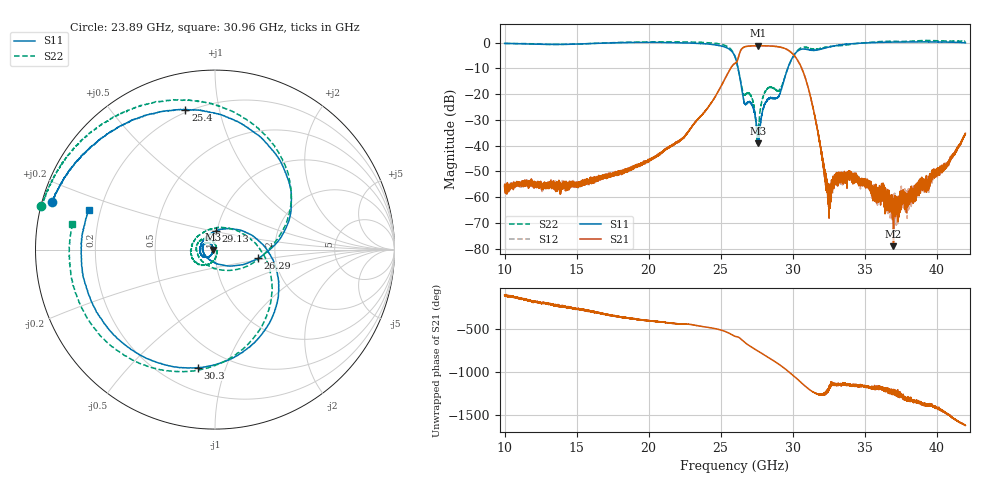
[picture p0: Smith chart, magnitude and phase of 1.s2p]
!The following data was pulled from an Agilent PNA
!This sNp file was generated from the data in the RF Test software
!NOTE:  Smoothing/Math/Corrections applied on any given trace ARE included in the data saved here
# MHz S dB R 50
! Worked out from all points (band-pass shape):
!   12801 points, 10 GHz to 42 GHz, reference 50 ohm
!   highest |S21| = -1.25 dB at 27.63 GHz (marker M1); lowest = -79.1 dB at 37.01 GHz (marker M2)
!   |S21| within 3 dB of the highest: 26.31 GHz to 29.98 GHz (3.668 GHz wide, 13 % of centre)
!   lowest |S11| = -39.2 dB at 27.63 GHz (marker M3), VSWR 1.02, Z = 48.9 - j0.0915 ohm
!   |S11| at or under -10 dB: 26.21 GHz to 29.66 GHz (3.449 GHz wide, 12.3 % of centre)
!   |S22| runs from -39.4 to 0.8 dB; largest |S21 - S12| = 0.0073
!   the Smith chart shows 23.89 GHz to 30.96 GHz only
!   S11 on the Smith chart (normalised r, x): 23.89 GHz: 0.03, +0.14; 25.4 GHz: 0.18, +0.79; 26.29 GHz: 1.62, -0.17; 29.13 GHz: 0.99, +0.21; 30.3 GHz: 0.34, -0.81; 30.96 GHz: 0.15, +0.15
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10000  -0.34 144.0  -56.36 -108.2  -56.17 -106.3  -0.36 144.1
12945  -0.73 74.5  -54.89 155.6  -55.10 153.8  -0.73 75.6
15335  -0.55 -9.8  -54.07 77.9  -54.62 84.4  -0.54 -9.2
17607.5  -0.09 -78.2  -51.10 15.2  -51.23 14.1  -0.05 -77.6
20667.5  0.03 -136.5  -43.44 -54.9  -43.69 -55.0  0.24 -135.3
23885  -0.49 163.8  -26.93 -116.1  -26.94 -116.5  -0.02 165.9
25400  -1.96 102.0  -13.01 -175.3  -13.00 -175.6  -1.36 103.0
26000  -5.47 37.2  -8.10 134.2  -8.10 134.0  -5.45 37.4
26292.5  -12.22 -11.5  -4.68 119.5  -4.67 119.1  -12.00 -11.3
27017.5  -22.99 160.6  -1.36 23.2  -1.38 22.9  -20.03 153.9
27627.5  -38.00 -176.0  -1.25 -39.6  -1.29 -40.0  -33.97 -54.5
27630  -39.16 -175.1  -1.28 -39.9  -1.27 -40.3  -33.79 -54.9
28317.5  -21.93 -156.2  -1.33 -109.4  -1.34 -109.7  -17.56 -151.0
29130  -19.75 87.8  -1.74 161.5  -1.74 161.1  -18.15 83.2
29672.5  -9.86 -8.6  -2.92 93.2  -2.90 92.8  -9.98 -17.9
30302.5  -3.54 -98.3  -6.47 3.8  -6.47 3.4  -3.33 -98.8
30962.5  -2.64 162.7  -15.17 -94.4  -15.17 -94.6  -1.85 169.9
31335  -3.04 108.1  -23.36 -141.1  -23.33 -140.7  -2.47 114.4
32512.5  -1.79 -2.7  -59.66 -114.7  -59.45 -115.6  -1.63 -4.7
36667.5  0.11 -97.9  -61.19 -120.4  -61.65 -142.5  0.50 -99.2
37005  0.16 -101.1  -79.07 -126.9  -61.61 -150.6  0.46 -103.1
42000  -0.13 -140.0  -35.27 -175.7  -35.55 -175.9  0.45 -145.3
